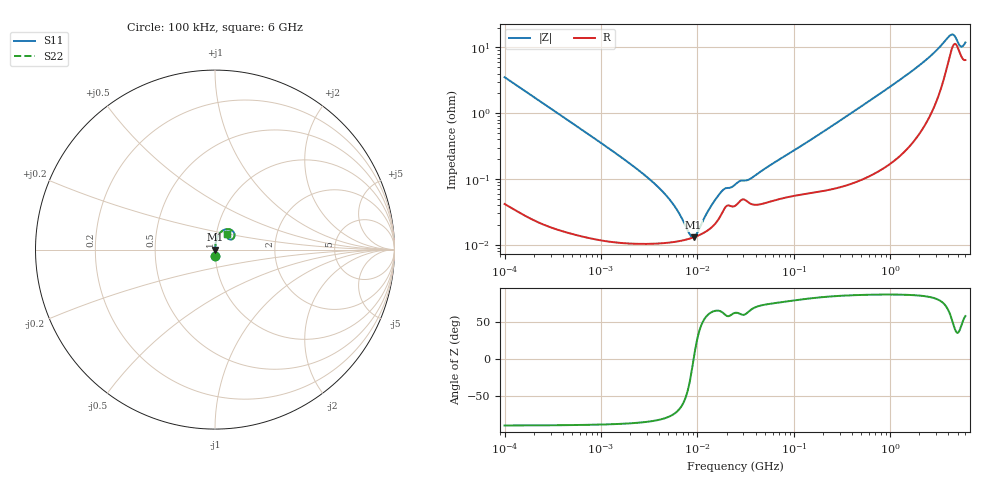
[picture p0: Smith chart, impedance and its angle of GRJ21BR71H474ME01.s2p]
!Murata Part Number: GRJ21BR71H474ME01
!These Parameters are Measured in Series Mode Connection
!Data Generated on Jun 19, 2026
!  o--ll--o
!Port1  Port2
!  o------o
!Operation Temp=25[degC], DC Bias Voltage=0[V]
!Freq. Start=100[kHz] Stop=6[GHz] 401[Steps]
# Hz S RI R 50
!Freq.(Hz) S11(Real) S11(Imag) S21(Real) S21(Imag) S12(Real) S12(Imag) S22(Real) S22(Imag)
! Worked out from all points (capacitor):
!   401 points, 100 kHz to 6 GHz, reference 50 ohm
!   read as one part in series: C = 449 nF near 105.7 kHz
!   lowest |Z| = 13 mohm at 9.1 MHz (marker M1)
!   series resonance near 9.128 MHz, so ESL is about 680 pH
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100000  0.00167 -0.0353  0.9983 0.0353  0.9983 0.0353  0.00167 -0.0353
631452  0.000166 -0.00563  0.9998 0.00563  0.9998 0.00563  0.000166 -0.00563
2060590  0.000107 -0.00165  0.9999 0.00165  0.9999 0.00165  0.000107 -0.00165
3987316  0.000106 -0.000728  0.9999 0.000728  0.9999 0.000728  0.000106 -0.000728
5701257  0.000111 -0.000384  0.9999 0.000384  0.9999 0.000384  0.000111 -0.000384
6724235  0.000115 -0.000245  0.9999 0.000245  0.9999 0.000245  0.000115 -0.000245
8151931  0.000123 -8.94e-05  0.9999 8.94e-05  0.9999 8.94e-05  0.000123 -8.94e-05
9100013  0.00013 -2.4e-06  0.9999 2.4e-06  0.9999 2.4e-06  0.00013 -2.4e-06
9882758  0.000136 6.3e-05  0.9999 -6.3e-05  0.9999 -6.3e-05  0.000136 6.3e-05
1.301164e7  0.000169 0.00029  0.9998 -0.00029  0.9998 -0.00029  0.000169 0.00029
1.713112e7  0.000267 0.000546  0.9997 -0.000546  0.9997 -0.000546  0.000267 0.000546
1.912349e7  0.000359 0.000615  0.9996 -0.000615  0.9996 -0.000615  0.000359 0.000615
2.517799e7  0.000403 0.00075  0.9996 -0.00075  0.9996 -0.00075  0.000403 0.00075
3.60007e7  0.000419 0.000938  0.9996 -0.000938  0.9996 -0.000938  0.000419 0.000938
1.546735e8  0.000633 0.00403  0.9994 -0.00403  0.9994 -0.00403  0.000633 0.00403
9.76689e8  0.00228 0.0247  0.9977 -0.0247  0.9977 -0.0247  0.00228 0.0247
2.229039e9  0.00978 0.0596  0.9902 -0.0596  0.9902 -0.0596  0.00978 0.0596
3.276068e9  0.0305 0.0956  0.9695 -0.0956  0.9695 -0.0956  0.0305 0.0956
4.082404e9  0.0786 0.1134  0.9214 -0.1134  0.9214 -0.1134  0.0786 0.1134
4.557193e9  0.1084 0.0858  0.8916 -0.0858  0.8916 -0.0858  0.1084 0.0858
5.374892e9  0.0749 0.0599  0.9251 -0.0599  0.9251 -0.0599  0.0749 0.0599
6e9  0.0688 0.0878  0.9312 -0.0878  0.9312 -0.0878  0.0688 0.0878
